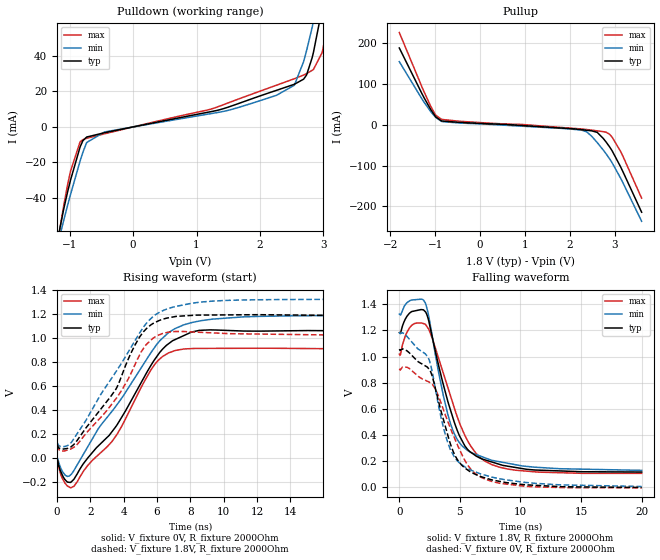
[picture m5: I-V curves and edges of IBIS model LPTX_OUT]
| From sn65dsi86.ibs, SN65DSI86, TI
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|   Model
[Model]   LPTX_OUT
Model_type   Output
Polarity   Non-Inverting
Vmeas = 0.9
Vref = 0
Cref = 1pF
Rref = 100000
|   typ   min   max
C_comp   1.494pF   1.437pF   1.561pF
[Voltage Range]   1.8   1.65   1.98
[Temperature Range]   27   125   -40
[Pullup Reference]   1.8   1.65   1.98
[Pulldown Reference]   -0   -0   -0
[Power Clamp Reference]   1.8   1.65   1.98
[GND Clamp Reference]   -0   -0   -0
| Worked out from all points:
|   slope of the pulldown table from 0 to 0.27 V, typ, clamps not added: 140 ohm
|   slope of the pullup table from 0 to 0.27 V, typ, clamps not added: 212 ohm
|   falling waveform, V_fixture 1.8V, R_fixture 2000Ohm: 20-80 % time 2.19ns typ, 1.92ns min, 2.34ns max; typ from 1.18 V to 0.116 V
|   rising waveform, V_fixture 0V, R_fixture 2000Ohm: 20-80 % time 2.75ns typ, 3.55ns min, 2.1ns max; typ from -0.003 V to 1.06 V
|   rising waveform, V_fixture 1.8V, R_fixture 2000Ohm: 20-80 % time 2.62ns typ, 3.2ns min, 2.59ns max; typ from 0.115 V to 1.19 V
|   falling waveform, V_fixture 0V, R_fixture 2000Ohm: 20-80 % time 2.07ns typ, 1.94ns min, 2.48ns max; typ from 1.06 V to -0.002 V
[Pulldown]
|   Voltage   I(typ)   I(min)   I(max)
-1.8V     -206mA     -193.6mA   -217mA
-1.152V   -56.96mA   -61.23mA   -57.2mA
-984.6mV  -29.88mA   -37.97mA   -24.86mA
-833.4mV  -11.16mA   -19.08mA   -8.288mA
-730.8mV  -5.694mA   -8.795mA   -6.408mA
2.261V    20.64mA    17.85mA    23.53mA
2.542V    24.06mA    23.52mA    27.18mA
2.731V    29.12mA    42.54mA    29.99mA
2.822V    39.07mA    56.18mA    31.92mA
2.979V    66.7mA     82.13mA    41.89mA
3.06V     83.11mA    96.33mA    56.58mA
3.595V    201.7mA    195.9mA    191.7mA
[Pullup]
|   Voltage   I(typ)   I(min)   I(max)
-1.8V     188.2mA    154.6mA    226.1mA
-1.292V   75.38mA    62.59mA    91.66mA
-1.098V   36.78mA    31.84mA    44.6mA
-990mV    19.47mA    17.99mA    23.54mA
-865.8mV  9.731mA    8.61mA     13.67mA
1.894V    -8.679mA   -9.444mA   -7.345mA
2.369V    -13.43mA   -17.12mA   -11.59mA
2.606V    -18.65mA   -43.71mA   -14.89mA
2.806V    -42.7mA    -71.62mA   -18.36mA
2.93V     -62.62mA   -91.97mA   -29.5mA
3.152V    -108.9mA   -136.4mA   -71.03mA
3.595V    -214.4mA   -236.7mA   -180mA
[Ramp]
R_load = 2000
|   typ   min   max
dV/dt_r   0.636568/2.72737e-09   0.71055/3.55276e-09   0.548172/2.09779e-09
dV/dt_f   0.640089/2.17661e-09   0.717611/1.92438e-09   0.547102/2.32916e-09
[Falling Waveform]
V_fixture = 1.8V
V_fixture_min = 1.65V
V_fixture_max = 1.98V
R_fixture = 2000Ohm
C_fixture = 0F
|   Time   V(typ)   V(min)   V(max)
0s        1.183V     1.325V     1.018V
1.023ns   1.344V     1.433V     1.239V
2.177ns   1.34V      1.402V     1.244V
2.728ns   1.146V     1.149V     1.137V
3.993ns   660.9mV    561mV      767mV
4.738ns   445.7mV    372.3mV    550.5mV
5.62ns    291.3mV    282.1mV    358.8mV
7.109ns   208.2mV    223.7mV    197.5mV
8.928ns   161.3mV    183.8mV    139.5mV
20ns      116.3mV    129.1mV    106.2mV
[Rising Waveform]
V_fixture = 0V
V_fixture_min = 0V
V_fixture_max = 0V
R_fixture = 2000Ohm
C_fixture = 0F
|   Time   V(typ)   V(min)   V(max)
0s        -2.763mV   5.02mV     -5.921mV
507.4ps   -181.6mV   -142.9mV   -211.5mV
1.023ns   -174.5mV   -101.4mV   -233.8mV
2.468ns   100.6mV    242.8mV    26.04mV
3.596ns   276.1mV    444.9mV    196.8mV
5.875ns   824.3mV    926mV      783.4mV
6.569ns   940.4mV    1.03V      866.7mV
7.597ns   1.021V     1.11V      909.3mV
11.13ns   1.059V     1.177V     915.4mV
20ns      1.058V     1.189V     907.7mV
[Rising Waveform]
V_fixture = 1.8V
V_fixture_min = 1.65V
V_fixture_max = 1.98V
R_fixture = 2000Ohm
C_fixture = 0F
|   Time   V(typ)   V(min)   V(max)
0s        115.4mV    128.5mV    105.2mV
182.1ps   81.72mV    99.94mV    64.48mV
632ps     81.37mV    105mV      68.07mV
1.221ns   149.5mV    205.7mV    116mV
3.537ns   574.6mV    719.3mV    494.5mV
4.953ns   1.008V     1.042V     858.1mV
5.729ns   1.119V     1.175V     995.1mV
6.407ns   1.16V      1.232V     1.041V
10.14ns   1.193V     1.314V     1.039V
20ns      1.185V     1.325V     1.02V
[Falling Waveform]
|Gnd
V_fixture = 0V
V_fixture_min = 0V
V_fixture_max = 0V
R_fixture = 2000Ohm
C_fixture = 0F
|   Time   V(typ)   V(min)   V(max)
0s        1.057V     1.185V     906.2mV
626ps     1.044V     1.154V     918.5mV
2.532ns   894mV      952.5mV    800mV
3.017ns   740.3mV    733.8mV    745.1mV
3.993ns   401mV      343.2mV    505.3mV
4.662ns   231.4mV    216.8mV    353.1mV
5.448ns   144.4mV    153mV      199.1mV
6.334ns   96.27mV    115.2mV    100.2mV
8.277ns   45.03mV    65mV       30.31mV
20ns      -1.746mV   5.613mV    -4.794mV
